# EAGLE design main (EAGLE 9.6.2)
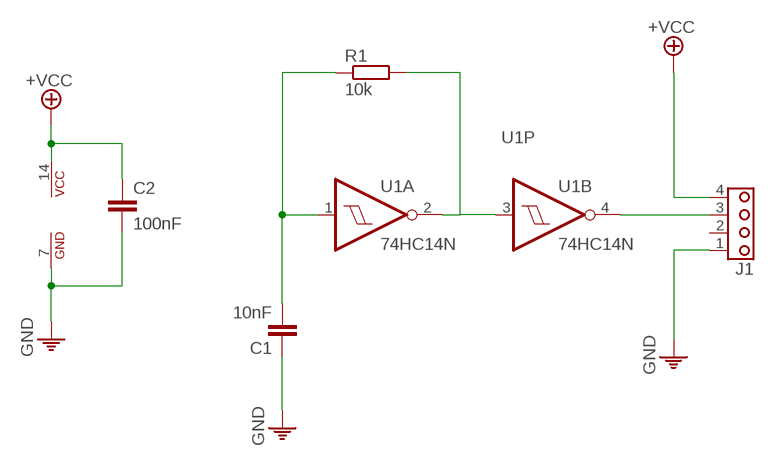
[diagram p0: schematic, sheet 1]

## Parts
C1  10nF  C-C2.5-2  [C2.5-2]
C2  100nF  C-C2.5-2  [C2.5-2]
J1  BORNIER_4-D4P  [MSTBA4]
R1  10k  R-CMS1206  [RCMS1206]
U1  74HC14N  [DIL14]

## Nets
GND: C1.1 C2.2 J1.1 U1.7(P:GND)
N$1: C1.2 R1.1 U1.1(A:I)
N$3: R1.2 U1.2(A:O) U1.3(B:I)
N$4: J1.3 U1.4(B:O)
VCC: C2.1 J1.4 U1.14(P:VCC) ; supply symbol labelled +VCC
Unconnected: J1.2 U1.5(C:I) U1.6(C:O) U1.8(D:O) U1.9(D:I) U1.10(E:O) U1.11(E:I) U1.12(F:O) U1.13(F:I)

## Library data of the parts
C1 C2 = 0IUT RLCQ:C: Condensateur non Polarisé, Symbole Européen; MAGASIN: (Armoire n°1)
J1 = 0IUT CONNECTEURS:BORNIER_4: BORNIER, 4 Contacts GEII/IUT ANGERS; MAGASIN: Bornier D4P (Armoire n°4) Bornier D4PF (Armoire n°4)
R1 = 0IUT RLCQ:R: Résistance Européenne; MAGASIN: (MAG-CMS)
U1 = 0IUT CI LOGIQUES:74HC14: 6 Portes INVERSEURS, Trigger de Schmitt Doc constructeur GEII/IUT ANGERS; MAGASIN: 74 HC 14 (Armoire n°4) KYT 14 (Armoire n°5)

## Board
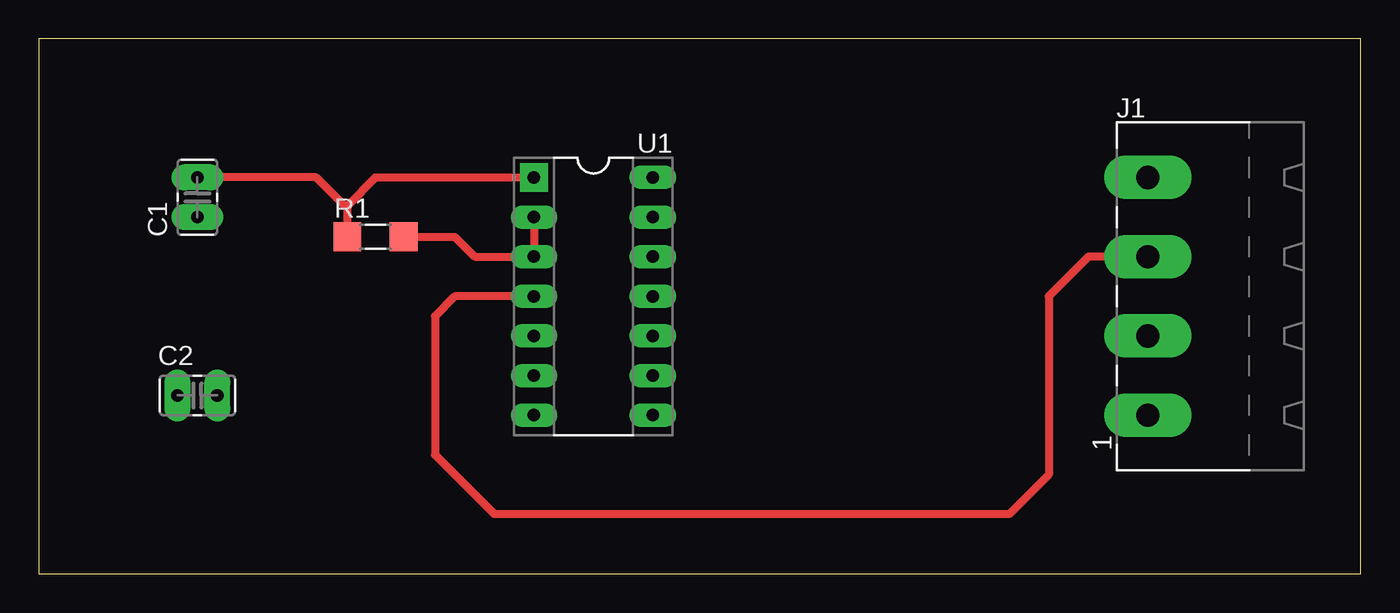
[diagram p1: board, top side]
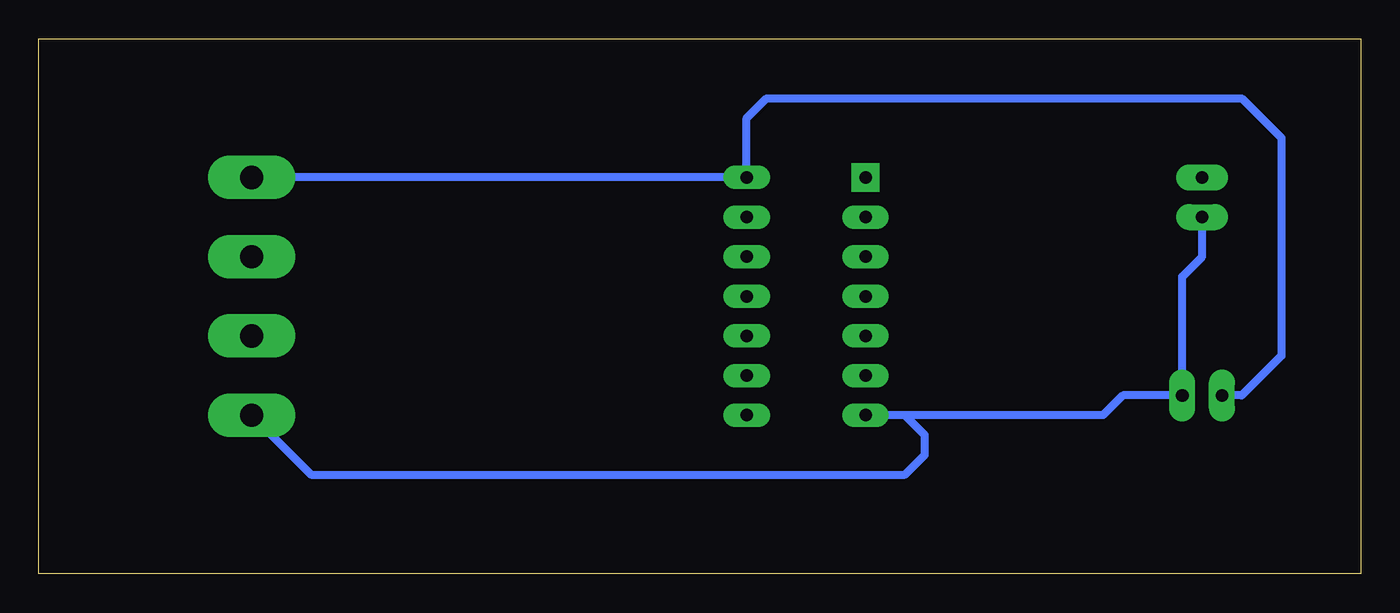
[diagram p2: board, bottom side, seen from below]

Size 84.76 x 34.28 mm. Coordinates in mm from the lower left corner, seen from the top.
Outline: 0,0 84.76,0 84.76,34.28 0,34.28 0,0
Copper layers (1*16): Top 0.105mm / dielectric 1.55mm / Bottom 0.105mm
Design rules "default": minimum track width 0.5mm, minimum drill 0.8mm, track to track 0.25mm, track to pad 0.25mm, pad to pad 0.25mm, via to via 0.25mm, smd to smd 0mil, copper to edge 0mil, drill to drill 0.35mm, minimum pad ring 0.25mm, minimum via ring 0.5mm, stop-mask expansion 0mil, vias tented up to drill 0.45mm, thermal gap 0.2mm

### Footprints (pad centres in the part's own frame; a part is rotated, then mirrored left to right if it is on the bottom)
C2.5-2 = drill 0.813 pad 1.676 long: 1 -1.27,0; 2 1.27,0
MSTBA4 = drill 1.499 pad 2.794 long: 1 -7.62,0; 2 -2.54,0; 3 2.54,0; 4 7.62,0
RCMS1206 = smd 1.778 x 1.854: 1 -1.803,0; 2 1.803,0
DIL14 = drill 0.8 pad 1.8 square: 1 -7.62,-3.81 | drill 0.8 pad 1.5 long: 2 -5.08,-3.81; 3 -2.54,-3.81; 4 0,-3.81; 5 2.54,-3.81; 6 5.08,-3.81; 7 7.62,-3.81; 8 7.62,3.81; 9 5.08,3.81; 10 2.54,3.81; 11 0,3.81; 12 -2.54,3.81; 13 -5.08,3.81; 14 -7.62,3.81

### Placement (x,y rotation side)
C1  10.16,24.13 90 top
C2  10.16,11.43 0 top
J1  71.12,17.78 90 top
R1  21.59,21.59 0 top
U1  35.56,17.78 270 top

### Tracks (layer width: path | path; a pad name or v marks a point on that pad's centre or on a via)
GND
  Bottom 0.5: J1.1 67.31,6.35 29.21,6.35 27.94,7.62 27.94,8.89 29.21,10.16 | 29.21,10.16 U1.7 | C1.1 10.16,20.32 11.43,19.05 C2.2 15.24,11.43 16.51,10.16 29.21,10.16
N$1
  Top 0.5: U1.1 21.59,25.4 19.79,23.6 19.79,23.39 | R1.1 19.79,23.39 | 19.79,23.39 17.78,25.4 C1.2
N$3
  Top 0.5: R1.2 26.67,21.59 27.94,20.32 U1.3 U1.2
N$4
  Top 0.5: U1.4 26.67,17.78 25.4,16.51 25.4,7.62 29.21,3.81 62.23,3.81 64.77,6.35 64.77,17.78 67.31,20.32 J1.3
VCC
  Bottom 0.5: J1.4 U1.14 39.37,29.21 38.1,30.48 7.62,30.48 5.08,27.94 5.08,13.97 7.62,11.43 C2.1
